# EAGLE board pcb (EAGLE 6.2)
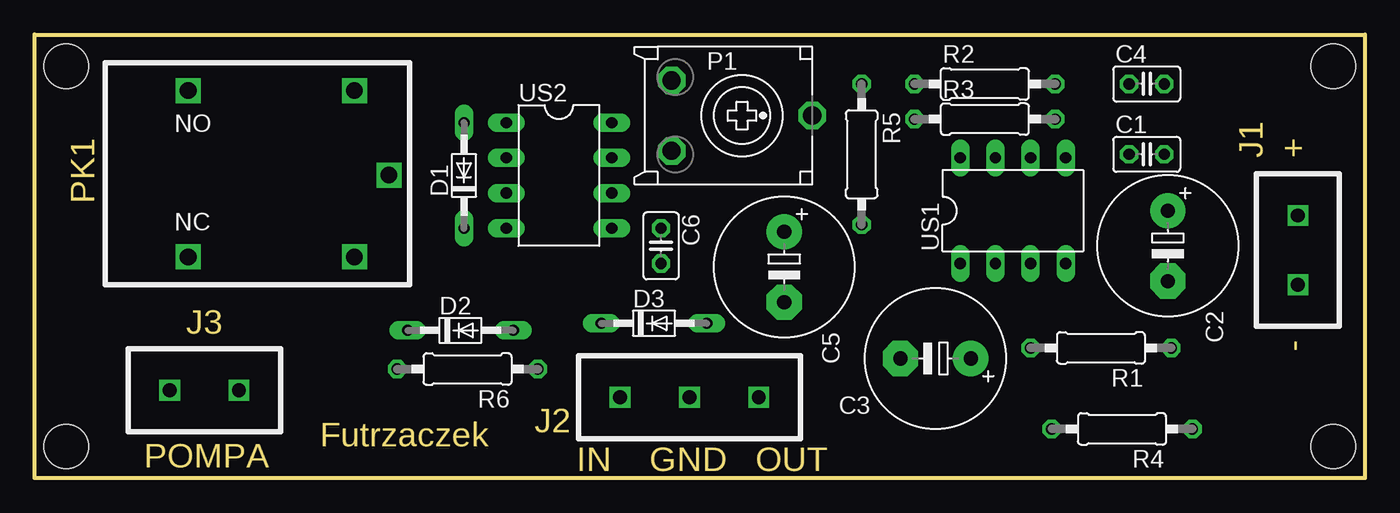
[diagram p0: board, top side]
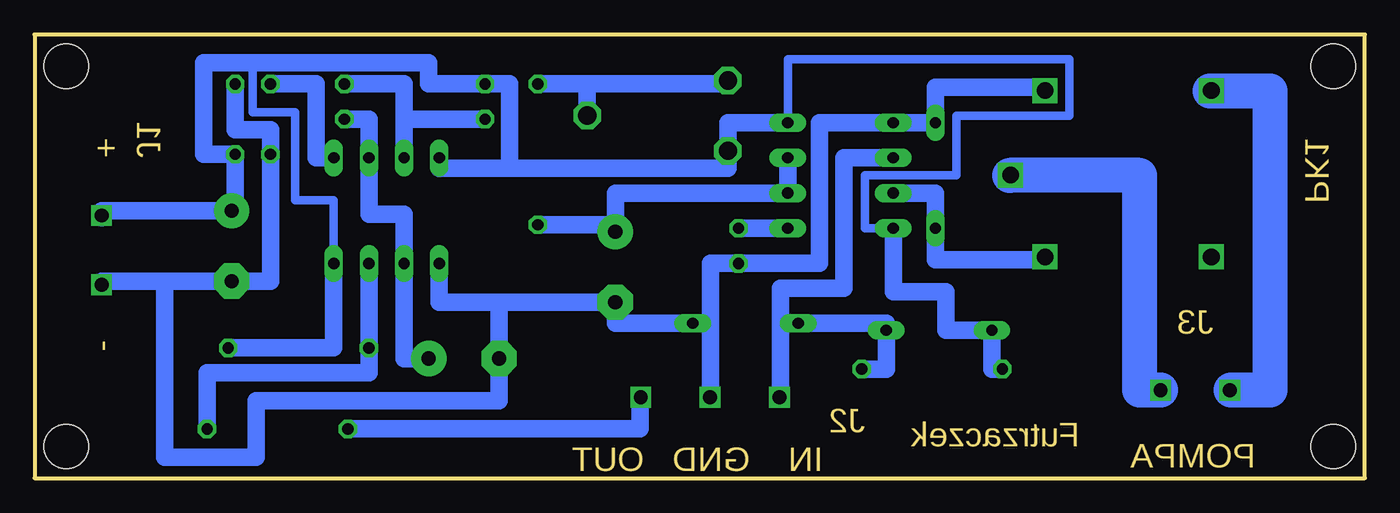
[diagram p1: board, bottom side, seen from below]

Size 96.01 x 32 mm. Coordinates in mm from the lower left corner, seen from the top.
Outline: 0,32 96.01,32 96.01,0 0,0 0,32
Copper layers (1*16): Top 0.035mm / dielectric 1.5mm / Bottom 0.035mm
Design rules: minimum track width 10mil, minimum drill 24mil, track to track 8mil, track to pad 8mil, pad to pad 8mil, via to via 8mil, smd to smd 8mil, copper to edge 40mil, drill to drill 8mil, minimum pad ring 10mil, minimum via ring 8mil, stop-mask expansion 4mil, vias tented up to drill 0mil, thermal gap 10mil
Holes 3.2 mm at 2.29,29.72 2.29,2.29 93.73,2.29 93.73,29.72

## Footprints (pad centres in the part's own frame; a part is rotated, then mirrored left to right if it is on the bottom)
C025-025X050 = drill 0.813 octagon: 1 -1.27,0; 2 1.27,0
E5-10,5 = drill 1.016 pad 2.54: + -2.54,0 | drill 1.016 pad 2.54 octagon: - 2.54,0
DO34-7 = drill 0.813 long: A 3.81,0; C -3.81,0
MOJA = drill 1.2 square: P$1 18,2; P$2 18,14; P$3 6,14; P$4 6,2; P$5 20.5,7.9
ECP10S = drill 1.321 octagon: A -2.54,-5.08; E 2.54,-5.08; S 0,5.08
0207/10 = drill 0.813 octagon: 1 -5.08,0; 2 5.08,0
DIL08 = drill 0.813 long: 1 -3.81,-3.81; 2 -1.27,-3.81; 3 1.27,-3.81; 4 3.81,-3.81; 5 3.81,3.81; 6 1.27,3.81; 7 -1.27,3.81; 8 -3.81,3.81

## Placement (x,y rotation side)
C1  [C025-025X050]  80.26,23.37 0 top
C2  [E5-10,5]  81.79,16.76 270 top
C3  [E5-10,5]  65.02,8.64 180 top
C4  [C025-025X050]  80.26,28.45 0 top
C5  [E5-10,5]  54.1,15.24 270 top
C6  [C025-025X050]  45.21,16.76 270 top
D1  [DO34-7]  30.99,21.84 90 top
D2  [DO34-7]  30.73,10.67 0 top
D3  [DO34-7]  44.7,11.18 0 top
E$2  [MOJA]  5.08,13.97 0 top
P1  [ECP10S]  51.05,26.16 270 top
R1  [0207/10]  76.96,9.4 180 top
R2  [0207/10]  68.58,28.45 0 top
R3  [0207/10]  68.58,25.91 0 top
R4  [0207/10]  78.49,3.56 180 top
R5  [0207/10]  59.69,23.37 270 top
R6  [0207/10]  31.24,7.87 180 top
US1  [DIL08]  70.61,19.3 0 top
US2  [DIL08]  37.85,21.84 270 top

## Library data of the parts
C1-C6 R1-R6 = rcl
D1-D3 = diode
E$2 = relay
P1 = pot
US1 US2 = 40xx

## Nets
S$7: US2.1
S$17: C6.1 US2.5
S$18: R4.2
S$19: US2.7
S$20: C1.1 C2.- C3.- C4.2 C5.- D3.A US1.1
S$21: D2.A D3.C R6.1 US2.2
S$22: D2.C P1.E R6.2 US2.4 US2.8
S$23: C5.+ R5.2 US2.6
S$24: P1.S R5.1
S$26: R1.1
S$27: US1.8
S$28: C3.+ R3.2 US1.2 US1.6
S$29: R3.1
S$30: R1.2 R4.1
S$31: C4.1 US1.5
S$32: C1.2 C2.+ R2.1

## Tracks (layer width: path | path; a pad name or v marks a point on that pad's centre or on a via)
S$1  (via drill 1)
  other vias: 14.74,6.35
S$2  (via drill 1)
  other vias: 9.74,6.35
S$3
  Bottom 2.54: 11.18,27.94 6.86,27.94 6.86,6.35 9.65,6.35
S$4  (via drill 1)
  other vias: 91.18,13.96
S$5  (via drill 1)
  other vias: 91.18,18.96
S$7
  Bottom 1.27: 23.11,28.19 30.99,28.19 30.99,25.65 US2.1 39.37,25.65 39.37,15.49 47.24,15.49 47.24,5.84
S$10
  Bottom 2.54: 14.73,6.35 16.26,6.35 16.26,21.84 25.65,21.84
S$12
  Bottom 1.27: 34.04,20.57 30.99,20.57 30.99,15.75 23.37,15.75 23.37,16 23.11,16
S$13  (via drill 1)
  other vias: 42.26,5.85
S$14  (via drill 1)
  other vias: 47.26,5.85
S$15  (via drill 1)
  other vias: 47.26,5.85
S$16  (via drill 1)
  other vias: 52.26,5.85
S$17
  Bottom 1.27: US2.5 C6.1
S$18
  Bottom 1.27: R4.2 52.32,3.56 52.32,5.84
S$19
  Bottom 1.27: US2.7 41.66,20.83
S$20
  Bottom 1.27: 47.5,11.18 D3.A 54.1,11.18 C5.- 62.48,12.7 | 91.19,13.97 91.19,14.22 86.61,14.22 | 62.48,12.7 66.8,12.7 US1.1 | 62.48,12.7 C3.- 62.48,5.59 80.01,5.59 80.01,1.52 86.61,1.52 86.61,14.22 | C4.2 81.53,25.15 78.99,25.15 C1.1 78.99,14.22 C2.- 86.61,14.22
S$21
  Bottom 1.27: US2.2 37.59,23.11 37.59,13.72 42.16,13.72 42.16,11.18 | 42.16,11.18 42.16,5.84 | 42.16,11.18 D3.C 34.54,11.18 D2.A 34.54,7.87 R6.1
S$22
  Bottom 0.61: US2.4 36.07,18.03 36.07,21.84 29.46,21.84 29.46,26.16 21.34,26.16 21.34,30.23 41.66,30.23 US2.8
  Bottom 1.27: R6.2 26.92,7.87 D2.C 30.23,10.67 30.23,13.46 34.04,13.46 US2.4 | US2.8 45.97,25.65 P1.E
S$23
  Bottom 1.27: US2.6 54.1,20.57 54.1,18.29 | 54.1,18.29 C5.+ | R5.2 54.1,18.29
S$24
  Bottom 1.27: 45.72,28.45 56.13,28.45 | 56.13,28.45 P1.S | R5.1 56.13,28.45
S$26
  Bottom 0.61: 74.42,15.75 74.42,20.07 77.22,20.07 77.22,26.42 80.26,26.42 80.26,29.72
  Bottom 1.27: R1.1 74.42,9.4 74.42,15.75 74.42,16
S$27
  Bottom 1.27: 45.97,23.37 45.97,22.35 66.8,22.35 US1.8
S$28
  Bottom 1.27: C3.+ 69.34,8.64 US1.2 69.34,19.05 71.88,19.05 US1.6 71.88,25.91 R3.2
S$29
  Bottom 1.27: R3.1 69.34,25.91 | 69.34,25.91 69.34,22.86 | 73.66,28.45 69.34,28.45 69.34,25.91
S$30
  Bottom 1.27: R4.1 83.57,7.62 71.88,7.62 R1.2 71.88,15.75
S$31
  Bottom 1.27: US1.5 75.69,23.11 75.69,28.45 C4.1
S$32
  Bottom 1.27: 61.72,22.61 61.72,28.45 R2.1 67.56,28.45 67.56,29.97 83.82,29.97 83.82,23.37 C1.2 81.53,19.3 C2.+ 91.19,19.3 91.19,18.8

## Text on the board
Dimension: J1 | + | PK1 | J3 | - | J2 | Futrzaczek | POMPA | IN GND OUT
